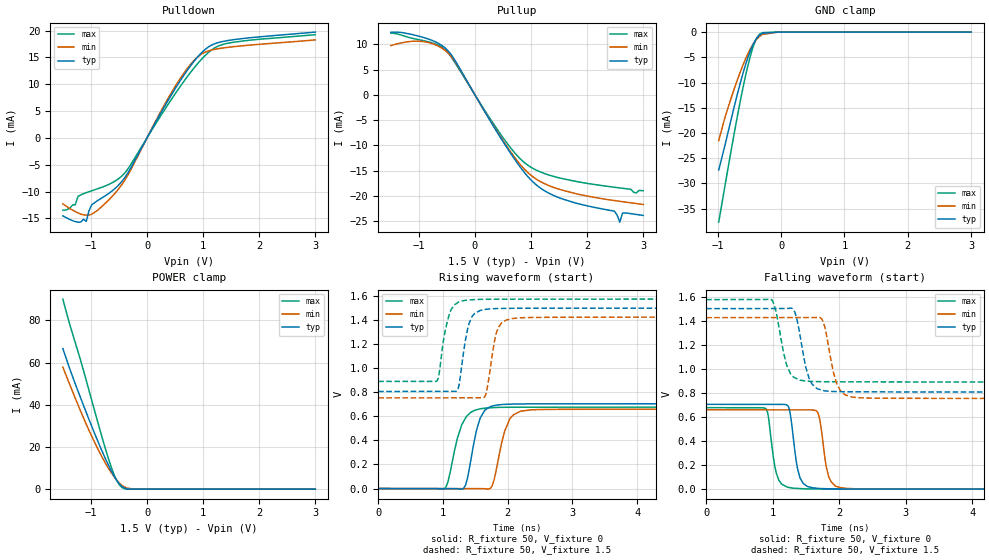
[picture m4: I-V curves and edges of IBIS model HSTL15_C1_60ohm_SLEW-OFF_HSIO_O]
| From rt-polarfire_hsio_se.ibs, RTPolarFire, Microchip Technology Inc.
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|   Model HSTL15_C1_60ohm_SLEW-OFF_HSIO_O
[Model]   HSTL15_C1_60ohm_SLEW-OFF_HSIO_O
Model_type   Output
Polarity   Non-Inverting
Enable   Active-High
Vmeas =   0.75
Cref =   5p
Rref =   50
Vref =   0.75
|   typ   min   max
C_comp_pullup   1.335e-12   1.335e-12   1.380e-12
C_comp_pulldown  1.335e-12   1.335e-12   1.380e-12
[Temperature Range]  25C   125C   -55C
[Voltage Range]  1.5   1.425   1.575
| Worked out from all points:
|   slope of the pulldown table from 0 to 0.225 V, typ, clamps not added: 52.7 ohm
|   slope of the pullup table from 0 to 0.225 V, typ, clamps not added: 52.8 ohm
|   GND clamp passes 1 mA (typ) near -0.37 V on its own axis
|   POWER clamp passes 1 mA (typ) near -0.43 V on its own axis
|   rising waveform, R_fixture 50, V_fixture 0: 20-80 % time 164ps typ, 178ps min, 191ps max; typ from 0 V to 0.705 V
|   rising waveform, R_fixture 50, V_fixture 1.5: 20-80 % time 125ps typ, 124ps min, 134ps max; typ from 0.807 V to 1.5 V
|   falling waveform, R_fixture 50, V_fixture 0: 20-80 % time 107ps typ, 106ps min, 104ps max; typ from 0.705 V to 0 V
|   falling waveform, R_fixture 50, V_fixture 1.5: 20-80 % time 151ps typ, 150ps min, 150ps max; typ from 1.5 V to 0.807 V
[GND Clamp]
| Voltage   I(typ)   I(min)   I(max)
-984.4mV  -27.37mA   -21.52mA   -37.7mA
-885.9mV  -22.43mA   -16.92mA   -30.48mA
-787.5mV  -17.27mA   -13.04mA   -23.4mA
-689.1mV  -12.26mA   -9.44mA    -16.62mA
-590.6mV  -7.7mA     -6.188mA   -10.38mA
-492.2mV  -3.93mA    -3.481mA   -5.066mA
-443mV    -2.467mA   -2.402mA   -2.955mA
-393.7mV  -1.355mA   -1.538mA   -1.375mA
-344.5mV  -621.9uA   -897uA     -448.3uA
-295.3mV  -232uA     -469.2uA   -100.1uA
-49.22mV  -334.5nA   -3.793uA   -95.68nA
3V        0A         0A         0A
[POWER Clamp]
| Voltage   I(typ)   I(min)   I(max)
-1.5V     66.64mA    57.8mA     90.1mA
-1.378V   57.06mA    49.6mA     78.07mA
-1.28V    49.9mA     43.13mA    69.49mA
-1.034V   32.99mA    27.83mA    46.7mA
-836.7mV  20.16mA    16.97mA    27.85mA
-689.1mV  11.42mA    9.956mA    14.55mA
-590.6mV  6.331mA    6.012mA    7.055mA
-541.4mV  4.184mA    4.318mA    4.125mA
-443mV    1.134mA    1.688mA    703.5uA
-344.5mV  93.53uA    432.5uA    21.45uA
-49.22mV  620.3nA    2.506uA    250nA
3V        0A         0A         0A
[Pullup]
| Voltage   I(typ)   I(min)   I(max)
-1.5V     12.36mA    9.717mA    12.19mA
-935.2mV  11.38mA    10.54mA    10.74mA
-492.2mV  8.849mA    8.399mA    8.457mA
609.4mV   -11.12mA   -10.84mA   -10.1mA
890.6mV   -15.47mA   -14.8mA    -13.48mA
1.172V    -18.46mA   -17.17mA   -15.27mA
1.795V    -21.39mA   -19.53mA   -17.1mA
2.484V    -22.99mA   -20.89mA   -18.26mA
2.583V    -25.17mA   -21.05mA   -18.4mA
2.632V    -23.36mA   -21.12mA   -18.47mA
2.878V    -23.64mA   -21.49mA   -19.38mA
3V        -23.84mA   -21.67mA   -18.96mA
[Pulldown]
| Voltage   I(typ)   I(min)   I(max)
-1.5V     -14.53mA   -12.3mA    -13.47mA
-1.28V    -15.61mA   -13.74mA   -12.46mA
-1.23V    -15.72mA   -14mA      -10.92mA
-1.083V   -15.56mA   -14.42mA   -10.21mA
-984.4mV  -12.45mA   -14.23mA   -9.857mA
-639.8mV  -10.03mA   -11.12mA   -8.463mA
-344.5mV  -6.581mA   -6.994mA   -5.838mA
609.4mV   10.93mA    11.35mA    9.846mA
843.8mV   14.35mA    14.5mA     13.11mA
1.078V    16.83mA    16.16mA    15.77mA
1.5V      18.24mA    16.95mA    17.76mA
3V        19.72mA    18.27mA    19.23mA
[Ramp]
dV/dt_r   0.422899/0.163829n  0.395776/0.178187n  0.40623/0.190688n
dV/dt_f   0.41579/0.151302n  0.402688/0.149868n  0.410802/0.149714n
R_load = 50
[Rising Waveform]
R_fixture = 50
V_fixture = 0
V_fixture_min = 0
V_fixture_max = 0
| Time   V(typ)   V(min)   V(max)
0s        1.706uV    3.25uV     2.624uV
1.017ns   -625.9uV   -471.9uV   -3.943mV
1.313ns   -2.092mV   -610.2uV   551.2mV
1.376ns   77.69mV    -639.6uV   605.5mV
1.577ns   587.7mV    -733.6uV   663.2mV
1.76ns    684.9mV    22.34mV    672.2mV
1.889ns   697.4mV    330.6mV    675mV
2.034ns   701.4mV    580mV      675.6mV
2.364ns   703.7mV    654.3mV    676.1mV
10ns      704.8mV    659.6mV    677.1mV
[Rising Waveform]
R_fixture = 50
V_fixture = 1.5
V_fixture_min = 1.425
V_fixture_max = 1.575
| Time   V(typ)   V(min)   V(max)
0s        807mV      753.8mV    890.3mV
907ps     807.6mV    754mV      894.5mV
1.069ns   807.7mV    754.1mV    1.39V
1.213ns   810.5mV    754.1mV    1.539V
1.255ns   879mV      754.1mV    1.553V
1.386ns   1.336V     754.2mV    1.567V
1.646ns   1.488V     763.5mV    1.573V
1.832ns   1.496V     1.304V     1.574V
2.066ns   1.498V     1.412V     1.574V
10ns      1.5V       1.425V     1.575V
[Falling Waveform]
R_fixture = 50
V_fixture = 0
V_fixture_min = 0
V_fixture_max = 0
| Time   V(typ)   V(min)   V(max)
0s        704.8mV    659.6mV    677mV
899ps     704.2mV    659.2mV    667.3mV
1.052ns   704.1mV    659.1mV    137.7mV
1.218ns   697.3mV    659mV      17.4mV
1.41ns    94mV       658.9mV    4.811mV
1.594ns   11.97mV    658mV      1.955mV
1.706ns   5.467mV    581.3mV    1.549mV
1.84ns    3.07mV     105.6mV    1.192mV
2.026ns   1.57mV     11.52mV    849.7uV
10ns      2.863uV    5.171uV    3.165uV
[Falling Waveform]
R_fixture = 50
V_fixture = 1.5
V_fixture_min = 1.425
V_fixture_max = 1.575
| Time   V(typ)   V(min)   V(max)
0s        1.5V       1.425V     1.575V
991ps     1.501V     1.426V     1.571V
1.209ns   1.501V     1.426V     1.032V
1.332ns   1.472V     1.426V     926mV
1.488ns   1.04V      1.426V     898.9mV
1.591ns   872.7mV    1.426V     895.1mV
1.741ns   822.8mV    1.411V     893.1mV
1.957ns   810.7mV    883.4mV    892.2mV
2.196ns   809mV      764.6mV    891.7mV
10ns      807mV      753.8mV    890.3mV
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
